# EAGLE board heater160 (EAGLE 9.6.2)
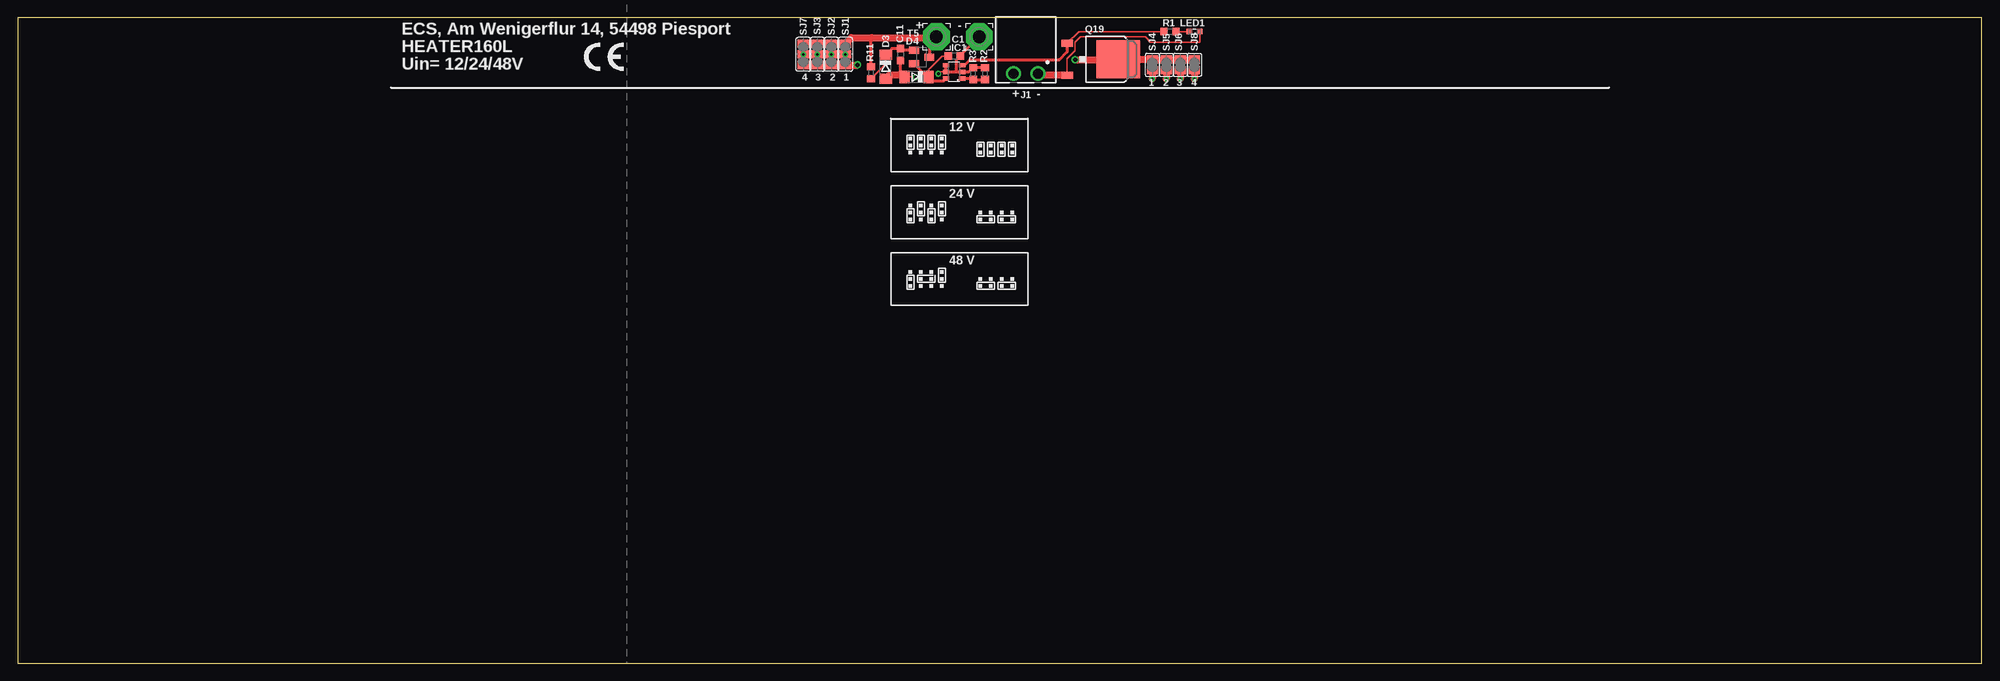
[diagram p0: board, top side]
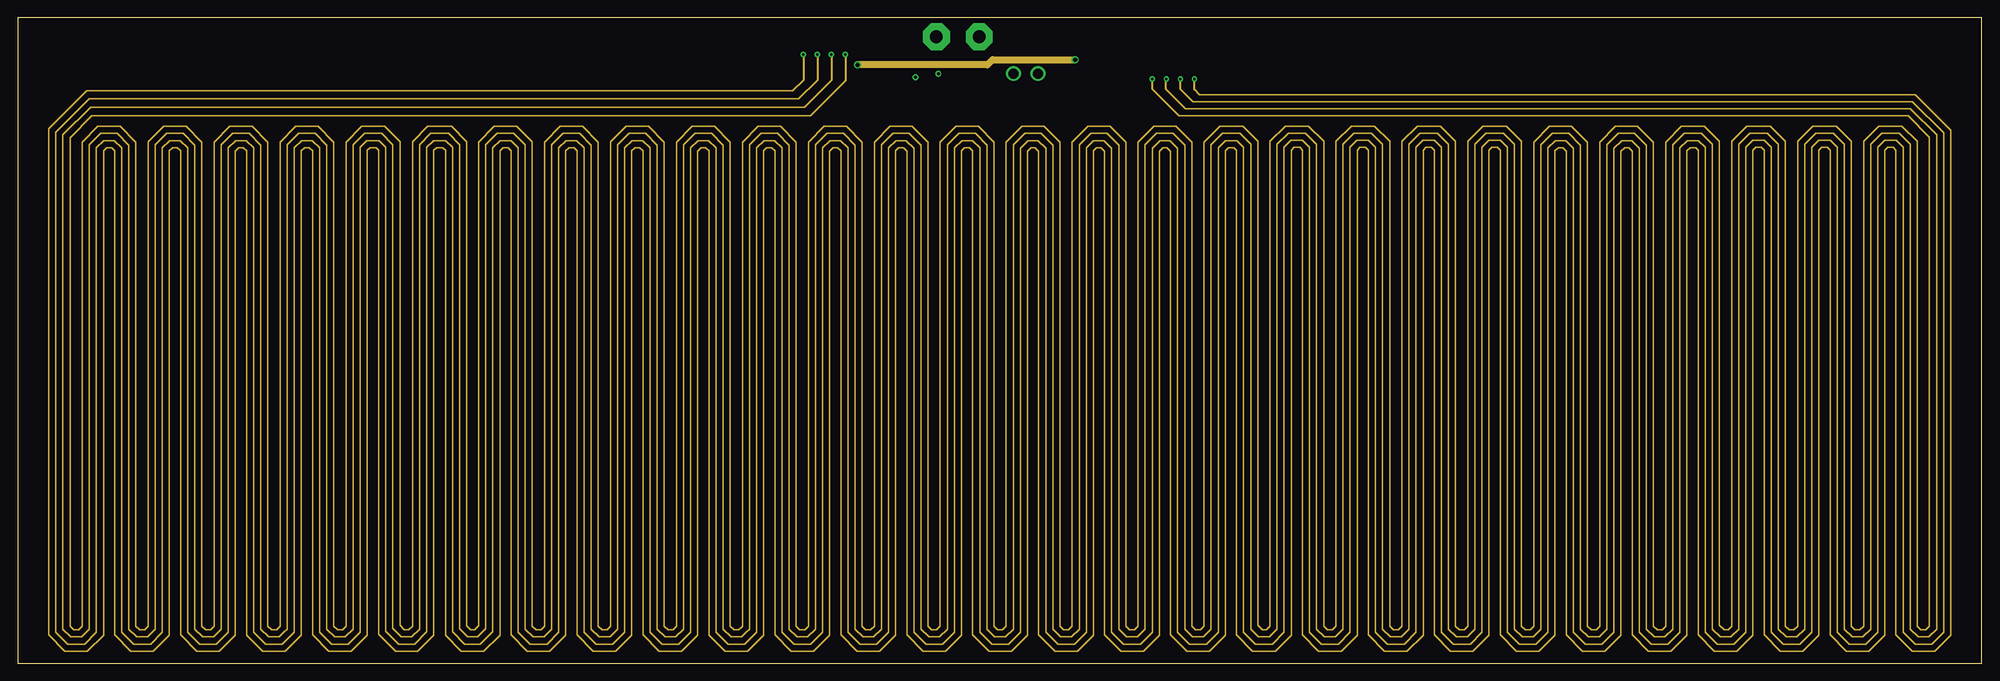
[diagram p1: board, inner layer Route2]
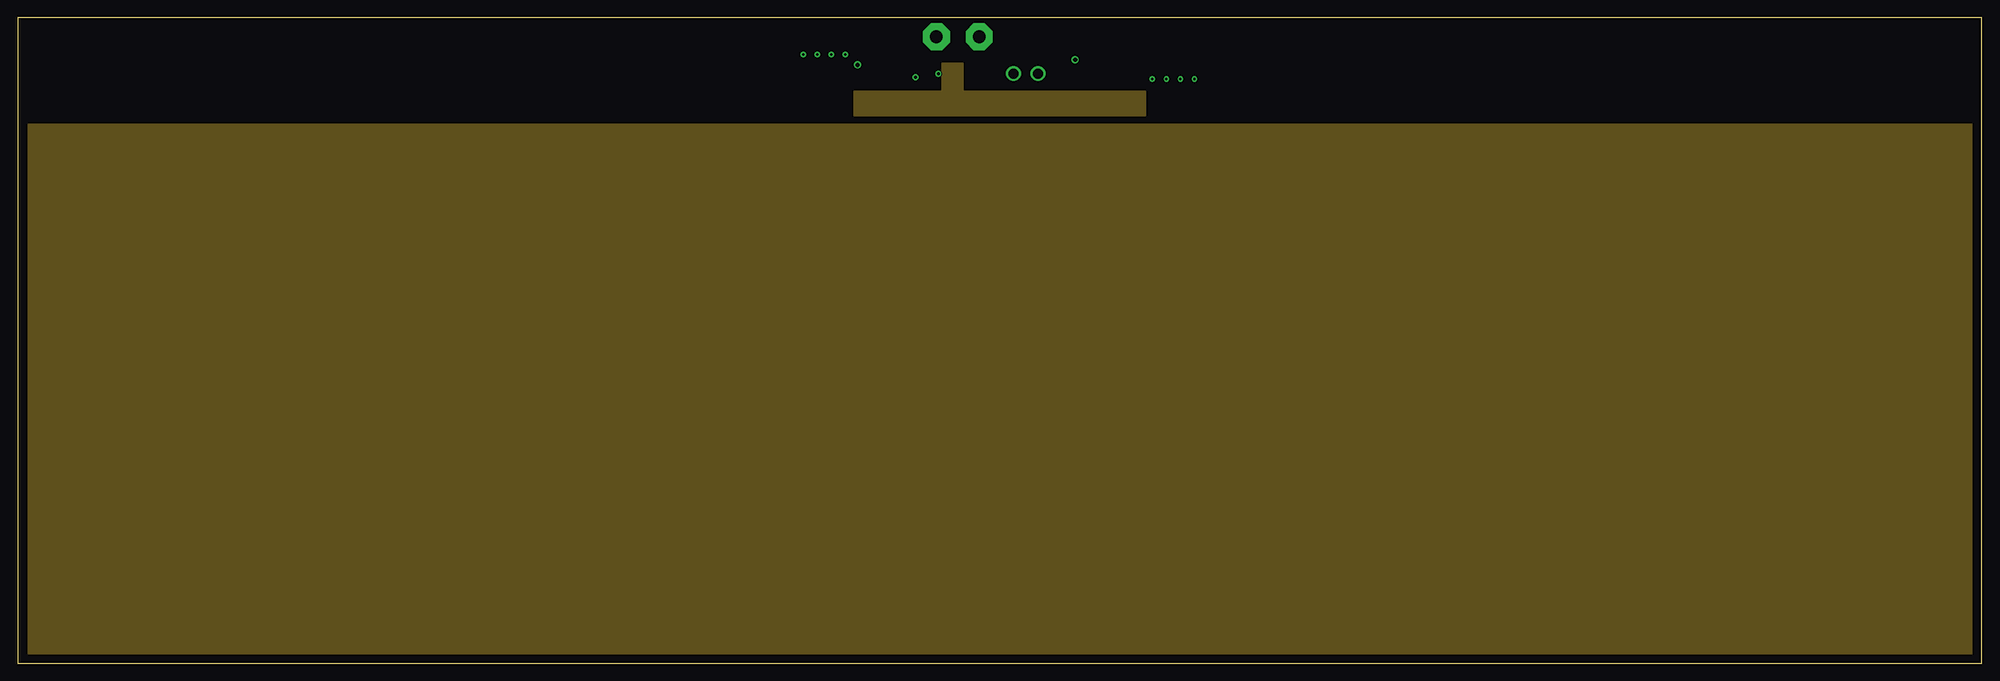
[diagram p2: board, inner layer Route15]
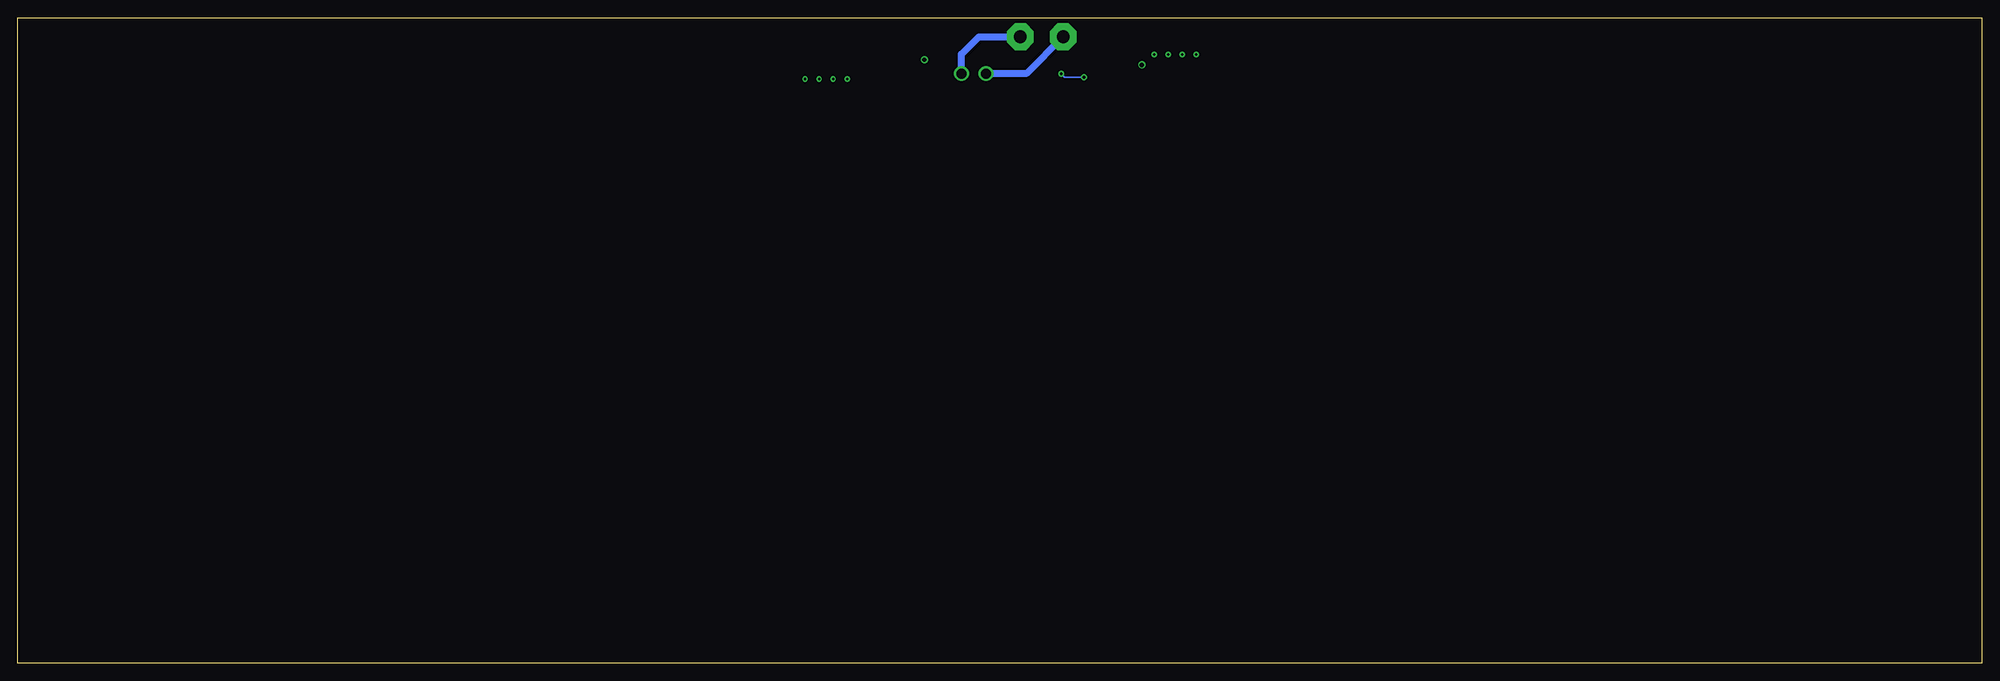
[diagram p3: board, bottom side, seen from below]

Size 280 x 92 mm. Coordinates in mm from the lower left corner, seen from the top.
Outline: 0,0 280,0 280,92 0,92 0,0
Copper layers (1+2*15+16): Top 0.035mm / dielectric 1.5mm / Route2 0.0175mm / dielectric 0.15mm / Route15 0.0175mm / dielectric 0.2mm / Bottom 0.035mm
Design rules "default *": minimum track width 6mil, minimum drill 0.35mm, track to track 6mil, track to pad 6mil, pad to pad 6mil, via to via 6mil, smd to smd 6mil, copper to edge 40mil, drill to drill 6mil, minimum pad ring 10mil, minimum via ring 8mil, stop-mask expansion 4mil, vias tented up to drill 0mil, thermal gap 10mil

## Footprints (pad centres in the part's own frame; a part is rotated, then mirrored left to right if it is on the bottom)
C0603 = smd 1.1 x 1: 1 -0.85,0; 2 0.85,0
SOD80C = smd 1.4 x 1.8: A 1.7,0; C -1.7,0
SOT23-6 = smd 0.6 x 0.9: 1 -0.95,-1.15; 2 0,-1.15; 3 0.95,-1.15; 4 0.95,1.15; 5 0,1.15; 6 -0.95,1.15
691322110002 = drill 1.4: 1 -1.75,0; 2 1.75,0
SML0603 = smd 0.8 x 0.8: A 0.75,0; C -0.75,0
3,81/1,4 = drill 1.8 pad 3.81 octagon: 1 0,0
D-PACK = smd 1 x 1.6: 1 -2.28,-4.8; 3 2.28,-4.8 | smd 5.4 x 6.2: 4 0,2.5
R0603 = smd 1 x 1.1: 1 -0.85,0; 2 0.85,0
SJ_2 = smd 1.168 x 1.6: 1 -1.524,0; 2 0,0; 3 1.524,0
SJ = smd 1.168 x 1.6: 1 -0.762,0; 2 0.762,0
SOT23-BEC = smd 1 x 1.4: B -0.95,-1.1; C 0,1.1; E 0.95,-1.1

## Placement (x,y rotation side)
C1  100n  [C0603]  133.52,86.52 0 top
C11  100n  [C0603]  125.85,86.73 270 top
D3  5V6  [SOD80C]  123.75,85 270 top
D4  5V1  [SOD80C]  128.13,83.55 180 top
IC1  MCP9510H  [SOT23-6]  133.5,84.25 90 top
J1  [691322110002]  143.71,84.01 180 top
LED1  [SML0603]  167.75,90 180 top
PAD1  [3,81/1,4]  130.97,89.26 0 top
PAD2  [3,81/1,4]  137.07,89.26 0 top
Q19  IRLR3110Z  [D-PACK]  154.41,86.05 270 top
R1  10k  [R0603]  164.25,90 180 top
R2  82k  [R0603]  137.89,84.02 270 top
R3  2M2  [R0603]  136.22,84.02 270 top
R11  100k  [R0603]  121.65,84.12 90 top
SJ1  [SJ_2]  118,86.75 90 top
SJ2  [SJ_2]  116,86.75 90 top
SJ3  [SJ_2]  114,86.75 90 top
SJ4  [SJ]  161.75,85.25 270 top
SJ5  [SJ]  163.75,85.25 270 top
SJ6  [SJ]  165.75,85.25 270 top
SJ7  [SJ_2]  112,86.75 90 top
SJ8  [SJ]  167.75,85.25 270 top
T5  BSR19A  [SOT23-BEC]  128.86,86.36 270 top
U$1  [CE-4MM]  80.75,84.38 0 top

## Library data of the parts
C1 C11 = rcl; PARTNO: C067; SPICEPREFIX: C
D3 = diode; PARTNO: D013
D4 = diode; PARTNO: D012
IC1 = mcp9509; PARTNO: IC333
J1 = Wurth_Connectors_WR-TBL Pluggable Connector; DATASHEET-URL: https://www.we-online.com/catalog/datasheet/691322110002.pdf; IR-UL: 10A; IR-VDE: 10.5A; MOUNT: THT; PART-NUMBER: 691322110002; PARTNO: CON212; PINS: 2; PITCH: 3.5mm; TYPE: Horizontal; WORKING-VOLTAGE-UL: 300V (AC); WORKING-VOLTAGE-VDE: 300V (AC)
LED1 = led; PARTNO: D078
PAD1 PAD2 = wirepad
Q19 = IRFR2607; PARTNO: T086
R1 = rcl; PARTNO: R221; SPICEPREFIX: R
R2 = rcl; PARTNO: R243; SPICEPREFIX: R
R3 = rcl; PARTNO: R277; SPICEPREFIX: R
R11 = rcl; PARTNO: R245; SPICEPREFIX: R
SJ1-SJ8 = jumper
T5 = transistor-neu-to92; PARTNO: T056
U$1 = logo

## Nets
+UB: J1.2 PAD1.1 R11.2 SJ1.3 SJ2.3 SJ3.3 SJ7.3 T5.C
GND: C1.2 C11.2 D3.A D4.A IC1.2 IC1.4 IC1.5 J1.1 LED1.C PAD2.1 Q19.3 R2.1 R3.1
N$1: IC1.3 Q19.1 R1.2
N$2: SJ1.2 SJ4.2
N$3: C11.1 D3.C R11.1 T5.B
N$4: IC1.1 R2.2 R3.2
N$5: C1.1 D4.C IC1.6 T5.E
N$6: LED1.A R1.1
N$7: SJ2.2 SJ5.2
N$8: SJ3.2 SJ6.2
N$9: SJ7.2 SJ8.2
N$11: Q19.4 SJ1.1 SJ2.1 SJ3.1 SJ4.1 SJ5.1 SJ6.1 SJ7.1 SJ8.1

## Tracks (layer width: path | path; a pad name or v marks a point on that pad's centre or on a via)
+UB
  Top 0.406: T5.C 130,86.4 130,88.29 130.85,89.14 PAD1.1 | R11.2 121.65,89.05 121.75,89.14
  Top 1.016: SJ7.3 SJ3.3 SJ2.3 SJ1.3 118.87,89.14 121.75,89.14 130.85,89.14
  Bottom 1.016: PAD1.1 136.22,84.01 J1.2
GND  (via drill 0.4)
  Top 0.2: LED1.C 168.5,88.5 161.5,88.5 160.75,89.25 151.5,89.25 150.75,88.5 150.75,87.25 149.61,86.11 Q19.3 | D4.A 127.95,83.55 v128,83.5 | v131.25,84 131.5,84.25 IC1.5
  Top 0.406: D4.A 125.85,84.13 C11.2 | 133.81,84.25 IC1.2 135.6,84.25 R3.1 R2.1 | 133.81,84.25 133.81,85.96 C1.2 134.37,86.56 PAD2.1 | IC1.4 IC1.5 133.81,84.25
  Top 1.016: D3.A 124.2,83.75 126.23,83.75 D4.A | Q19.3 145.7,83.77 J1.1
  Bottom 0.2: v128,83.5 130.75,83.5 v131.25,84
  Bottom 1.016: J1.1 145.46,86.79 142.99,89.26 PAD2.1
N$1
  Top 0.2: Q19.1 151.28,90 R1.2
  Top 0.406: IC1.3 134.95,85.2 135.75,86 148.5,86 149.61,87.11 Q19.1
N$2  (via drill 0.35, 0.35 pad 0.21)
  Top 1.016: SJ4.2 v161.75,83.25
  Route2 0.2: 118,83.02 113.04,78 10.61,78 7.48,74.87 7.48,5.27 8.01,4.75 8.71,4.75 9.22,5.25 9.22,74.26 11.45,76.49 14.64,76.49 16.88,74.25 16.88,5.27 17.4,4.75 18.11,4.75 18.62,5.25 18.62,74.27 20.84,76.49 24.04,76.49 26.28,74.25 26.28,5.27 26.8,4.75 27.51,4.75 28.02,5.25 28.02,74.26 30.25,76.49 33.44,76.49 35.68,74.25 35.68,5.27 36.2,4.75 36.9,4.75 37.2,5.05 37.42,5.27 37.42,74.26 39.65,76.49 42.84,76.49 45.08,74.25 45.08,5.27 45.6,4.75 46.32,4.75 46.82,5.25 46.82,74.26 49.05,76.49 52.31,76.49 54.5,74.3 54.5,5.37 55.12,4.76 55.76,4.76 56.29,5.28 56.29,74.32 58.46,76.49 61.84,76.49 64.01,74.32 64.01,5.32 64.59,4.75 65.13,4.75 65.72,5.34 65.72,74.26 67.95,76.49 71.16,76.49 73.38,74.27 73.38,5.27 73.91,4.75 74.61,4.75 75.12,5.25 75.12,74.26 77.35,76.49 80.54,76.49 82.78,74.25 82.78,5.27 83.3,4.75 84.01,4.75 84.52,5.25 84.52,74.27 86.74,76.49 89.94,76.49 92.18,74.25 92.18,5.27 92.7,4.75 93.41,4.75 93.92,5.25 93.92,74.26 96.15,76.49 99.34,76.49 101.58,74.25 101.58,5.27 102.1,4.75 102.8,4.75 103.1,5.05 103.32,5.27 103.32,74.26 105.55,76.49 108.74,76.49 110.98,74.25 110.98,5.27 111.5,4.75 112.22,4.75 112.72,5.25 112.72,74.26 114.95,76.49 118.14,76.49 120.38,74.25 120.38,5.27 120.91,4.75 121.61,4.75 122.12,5.25 122.12,74.26 124.35,76.49 127.5,76.49 129.78,74.22 129.78,5.27 130.31,4.75 131.01,4.75 131.52,5.25 131.52,74.26 133.75,76.49 136.94,76.49 139.18,74.25 139.18,5.27 139.71,4.75 140.41,4.75 140.92,5.25 140.92,74.26 143.15,76.49 146.31,76.49 148.58,74.22 148.58,5.27 149.1,4.75 149.82,4.75 150.32,5.25 150.32,74.26 152.55,76.49 155.71,76.49 157.98,74.22 157.98,5.27 158.5,4.75 159.21,4.75 159.72,5.25 159.72,74.26 161.95,76.49 165.1,76.49 167.38,74.22 167.38,5.27 167.91,4.75 168.61,4.75 169.12,5.25 169.12,74.26 171.35,76.49 174.64,76.49 176.78,74.36 176.78,5.42 177.45,4.75 178.01,4.75 178.52,5.25 178.52,74.36 180.69,76.53 184,76.53 186.18,74.36 186.18,5.27 186.71,4.75 187.41,4.75 187.92,5.25 187.92,74.36 190.09,76.53 193.41,76.53 195.58,74.36 195.58,5.27 196.1,4.75 196.81,4.75 197.32,5.25 197.32,74.36 199.5,76.53 202.81,76.53 204.98,74.36 204.98,5.27 205.5,4.75 206.21,4.75 206.72,5.25 206.72,74.36 208.9,76.53 212.21,76.53 214.38,74.36 214.38,5.27 214.91,4.75 215.61,4.75 216.12,5.25 216.12,74.26 218.35,76.49 221.5,76.49 223.78,74.22 223.78,5.27 224.31,4.75 225.01,4.75 225.52,5.25 225.52,74.26 227.75,76.49 230.91,76.49 233.18,74.22 233.18,5.27 233.71,4.75 234.41,4.75 234.92,5.25 234.92,74.26 237.15,76.49 240.44,76.49 242.58,74.36 242.58,5.42 243.25,4.75 243.81,4.75 244.32,5.25 244.32,74.36 246.5,76.53 249.81,76.53 251.98,74.36 251.98,5.27 252.5,4.75 253.21,4.75 253.72,5.25 253.72,74.36 255.9,76.53 259.2,76.53 261.38,74.36 261.38,5.27 261.9,4.75 262.61,4.75 263.12,5.25 263.12,74.36 265.3,76.53 268.61,76.53 270.78,74.36 270.78,5.27 271.31,4.75 272.01,4.75 272.52,5.25 272.52,74.95 269.48,78 165.55,78 161.75,81.8
  Route2 0.254: SJ1.2 118,83.02 | 161.75,81.8 v161.75,83.25
  other vias: 118,86.75
N$3
  Top 0.2: R11.1 123.75,85.37 D3.C
  Top 0.406: D3.C 124.63,87.58 C11.1 126.12,87.31 T5.B
N$4
  Top 0.406: IC1.1 136.22,83.3 R3.2 R2.2
N$5
  Top 0.2: C1.1 132.65,86.5 131.75,86.5 129.83,84.58 D4.C
  Top 0.406: T5.E 129.62,83.55 D4.C 130.08,83.3 130.2,83.3 130.5,83 132.02,83 IC1.6
N$6
  Top 0.2: R1.1 LED1.A
N$7  (via drill 0.35, 0.35 pad 0.21)
  Top 1.016: SJ5.2 v163.75,83.25
  Route2 0.2: 116,83.05 112.15,79.2 10.4,79.2 6.47,75.27 6.47,4.85 7.59,3.73 9.13,3.73 10.23,4.84 10.23,73.84 11.87,75.48 14.23,75.48 15.87,73.84 15.87,4.85 16.99,3.74 18.53,3.74 19.63,4.84 19.63,73.85 21.26,75.48 23.62,75.48 25.27,73.84 25.27,4.85 26.39,3.73 27.93,3.73 29.03,4.84 29.03,73.84 30.67,75.48 33.02,75.48 34.67,73.84 34.67,4.85 35.78,3.73 37.32,3.73 37.97,4.38 38.43,4.85 38.43,73.84 40.07,75.48 42.42,75.48 44.07,73.84 44.07,4.85 45.19,3.73 46.73,3.73 47.83,4.84 47.83,73.84 49.47,75.48 51.91,75.48 53.49,73.9 53.49,4.95 54.7,3.75 56.18,3.75 57.3,4.86 57.3,73.9 58.88,75.48 61.42,75.48 63.01,73.9 63.01,4.9 64.17,3.73 65.55,3.73 66.73,4.92 66.73,73.84 68.37,75.48 70.74,75.48 72.37,73.85 72.37,4.85 73.49,3.73 75.03,3.73 76.13,4.84 76.13,73.84 77.77,75.48 80.13,75.48 81.77,73.84 81.77,4.85 82.89,3.74 84.43,3.74 85.53,4.84 85.53,73.85 87.16,75.48 89.52,75.48 91.17,73.84 91.17,4.85 92.29,3.73 93.83,3.73 94.93,4.84 94.93,73.84 96.57,75.48 98.92,75.48 100.57,73.84 100.57,4.85 101.68,3.73 103.22,3.73 103.87,4.38 104.33,4.85 104.33,73.84 105.97,75.48 108.32,75.48 109.97,73.84 109.97,4.85 111.09,3.73 112.63,3.73 113.73,4.84 113.73,73.84 115.37,75.48 117.72,75.48 119.37,73.84 119.37,4.85 120.49,3.73 122.03,3.73 123.13,4.84 123.13,73.84 124.77,75.48 127.09,75.48 128.77,73.8 128.77,4.85 129.89,3.73 131.43,3.73 132.53,4.84 132.53,73.84 134.17,75.48 136.52,75.48 138.17,73.84 138.17,4.85 139.29,3.73 140.83,3.73 141.93,4.84 141.93,73.84 143.57,75.48 145.89,75.48 147.57,73.8 147.57,4.85 148.69,3.73 150.23,3.73 151.33,4.84 151.33,73.84 152.97,75.48 155.29,75.48 156.97,73.8 156.97,4.85 158.09,3.73 159.63,3.73 160.73,4.84 160.73,73.84 162.37,75.48 164.69,75.48 166.37,73.8 166.37,4.85 167.49,3.73 169.03,3.73 170.13,4.84 170.13,73.84 171.77,75.48 174.22,75.48 175.77,73.94 175.77,4.85 176.89,3.73 178.43,3.73 179.53,4.84 179.53,73.94 181.11,75.52 183.59,75.52 185.17,73.94 185.17,4.85 186.29,3.73 187.83,3.73 188.93,4.84 188.93,73.94 190.51,75.52 192.99,75.52 194.57,73.94 194.57,4.85 195.69,3.73 197.23,3.73 198.33,4.84 198.33,73.94 199.91,75.52 202.39,75.52 203.97,73.94 203.97,4.85 205.09,3.73 206.63,3.73 207.73,4.84 207.73,73.94 209.31,75.52 211.79,75.52 213.37,73.94 213.37,4.85 214.49,3.73 216.03,3.73 217.13,4.84 217.13,73.84 218.77,75.48 221.09,75.48 222.77,73.8 222.77,4.85 223.89,3.73 225.43,3.73 226.53,4.84 226.53,73.84 228.17,75.48 230.49,75.48 232.17,73.8 232.17,4.85 233.29,3.73 234.83,3.73 235.93,4.84 235.93,73.84 237.57,75.48 240.02,75.48 241.57,73.94 241.57,4.85 242.69,3.73 244.23,3.73 245.33,4.84 245.33,73.94 246.91,75.52 249.39,75.52 250.97,73.94 250.97,4.85 252.09,3.73 253.63,3.73 254.73,4.84 254.73,73.94 256.31,75.52 258.79,75.52 260.37,73.94 260.37,4.85 261.49,3.73 263.03,3.73 264.13,4.84 264.13,73.94 265.71,75.52 268.19,75.52 269.77,73.94 269.77,4.85 270.89,3.73 272.43,3.73 273.53,4.84 273.53,75.27 269.79,79.01 166.47,79.01 163.71,81.76
  Route2 0.254: SJ2.2 116,83.05 | 163.71,81.76 163.71,83.21
  Route2 0.4: 163.71,83.21 v163.75,83.25
  other vias: 116,86.75
N$8  (via drill 0.35, 0.35 pad 0.21)
  Top 1.016: SJ6.2 v165.75,83.25
  Route2 0.2: 114,83.05 111.35,80.4 10.2,80.4 5.46,75.66 5.46,4.43 7.17,2.73 9.55,2.73 11.24,4.42 11.24,73.43 12.28,74.47 13.81,74.47 14.86,73.42 14.86,4.43 16.57,2.73 18.95,2.73 20.64,4.42 20.64,73.44 21.68,74.47 23.21,74.47 24.26,73.42 24.26,4.43 25.97,2.73 28.35,2.73 30.04,4.42 30.04,73.43 31.09,74.47 32.61,74.47 33.66,73.42 33.66,4.43 35.37,2.73 37.73,2.73 39.44,4.43 39.44,73.43 40.49,74.47 42.01,74.47 43.06,73.42 43.06,4.43 44.77,2.73 47.15,2.73 48.84,4.42 48.84,73.53 49.79,74.47 51.51,74.47 52.48,73.5 52.48,4.53 54.29,2.73 56.59,2.73 58.3,4.45 58.3,73.48 59.29,74.47 61.01,74.47 61.99,73.48 61.99,4.48 63.75,2.73 65.97,2.73 67.74,4.5 67.74,73.43 68.79,74.47 70.32,74.47 71.36,73.44 71.36,4.43 73.07,2.73 75.45,2.73 77.14,4.42 77.14,73.43 78.18,74.47 79.71,74.47 80.76,73.42 80.76,4.43 82.47,2.73 84.85,2.73 86.54,4.42 86.54,73.44 87.58,74.47 89.11,74.47 90.16,73.42 90.16,4.43 91.87,2.73 94.25,2.73 95.94,4.42 95.94,73.43 96.99,74.47 98.51,74.47 99.56,73.42 99.56,4.43 101.27,2.73 103.63,2.73 105.34,4.43 105.34,73.43 106.39,74.47 107.91,74.47 108.96,73.42 108.96,4.43 110.67,2.73 113.05,2.73 114.74,4.42 114.74,73.43 115.79,74.47 117.31,74.47 118.36,73.42 118.36,4.43 120.07,2.73 122.45,2.73 124.14,4.42 124.14,73.43 125.19,74.47 126.67,74.47 127.76,73.38 127.76,4.43 129.47,2.73 131.85,2.73 133.54,4.42 133.54,73.43 134.59,74.47 136.11,74.47 137.16,73.42 137.16,4.43 138.87,2.73 141.25,2.73 142.94,4.42 142.94,73.36 144.05,74.47 145.47,74.47 146.56,73.38 146.56,4.43 148.27,2.73 150.65,2.73 152.34,4.42 152.34,73.43 153.39,74.47 154.87,74.47 155.96,73.38 155.96,4.43 157.67,2.73 160.05,2.73 161.74,4.42 161.74,73.36 162.85,74.47 164.27,74.47 165.36,73.38 165.36,4.43 167.07,2.73 169.45,2.73 171.14,4.42 171.14,73.43 172.19,74.47 173.81,74.47 174.76,73.52 174.76,4.43 176.47,2.73 178.85,2.73 180.54,4.42 180.54,73.52 181.53,74.51 183.17,74.51 184.16,73.52 184.16,4.43 185.87,2.73 188.25,2.73 189.94,4.42 189.94,73.52 190.93,74.51 192.57,74.51 193.56,73.52 193.56,4.43 195.27,2.73 197.65,2.73 199.34,4.42 199.34,73.52 200.33,74.51 201.97,74.51 202.96,73.52 202.96,4.43 204.67,2.73 207.05,2.73 208.74,4.42 208.74,73.52 209.73,74.51 211.37,74.51 212.36,73.52 212.36,4.43 214.07,2.73 216.45,2.73 218.14,4.42 218.14,73.43 219.19,74.47 220.67,74.47 221.76,73.38 221.76,4.43 223.47,2.73 225.85,2.73 227.54,4.42 227.54,73.36 228.65,74.47 230.07,74.47 231.16,73.38 231.16,4.43 232.87,2.73 235.25,2.73 236.94,4.42 236.94,73.43 237.99,74.47 239.61,74.47 240.56,73.52 240.56,4.43 242.27,2.73 244.65,2.73 246.34,4.42 246.34,73.52 247.33,74.51 248.97,74.51 249.96,73.52 249.96,4.43 251.67,2.73 254.05,2.73 255.74,4.42 255.74,73.52 256.73,74.51 258.37,74.51 259.36,73.52 259.36,4.43 261.07,2.73 263.45,2.73 265.14,4.42 265.14,73.52 266.13,74.51 267.77,74.51 268.76,73.52 268.76,4.43 270.47,2.73 272.85,2.73 274.54,4.42 274.54,75.56 270.08,80.02 167.53,80.02 165.75,81.8
  Route2 0.254: SJ3.2 114,83.05 | 165.75,81.8 v165.75,83.25
  other vias: 114,86.75
N$9  (via drill 0.35, 0.35 pad 0.21)
  Top 1.016: SJ8.2 v167.75,83.25
  Route2 0.2: 112,83.05 110.5,81.55 9.85,81.55 4.45,76.15 4.45,4.02 6.75,1.72 9.97,1.72 12.25,4 12.25,73.01 12.7,73.45 13.4,73.45 13.85,73 13.85,4.02 16.15,1.72 19.37,1.72 21.65,4 21.65,73.02 22.09,73.46 22.79,73.46 23.25,73 23.25,4.02 25.55,1.72 28.77,1.72 31.05,4 31.05,72.96 31.55,73.46 32.19,73.46 32.65,73 32.65,4 34.95,1.72 38.15,1.72 40.45,4 40.45,73.01 40.9,73.45 41.6,73.45 42.05,73 42.05,4.02 44.35,1.72 47.57,1.72 49.85,4 49.85,73.06 50.25,73.46 51.11,73.46 51.48,73.1 51.48,4.12 53.88,1.72 57.04,1.72 59.31,3.99 59.31,73.06 59.71,73.46 60.59,73.46 60.99,73.06 60.99,3.98 63.25,1.72 66.47,1.72 68.75,4 68.75,73.01 69.2,73.45 69.91,73.45 70.35,73.02 70.35,4.02 72.65,1.72 75.87,1.72 78.15,4 78.15,73.01 78.6,73.45 79.3,73.45 79.75,73 79.75,4.02 82.05,1.72 85.27,1.72 87.55,4 87.55,73.02 87.99,73.46 88.69,73.46 89.15,73 89.15,4.02 91.45,1.72 94.67,1.72 96.95,4 96.95,72.96 97.45,73.46 98.09,73.46 98.55,73 98.55,4 100.85,1.72 104.05,1.72 106.35,4 106.35,73.01 106.8,73.45 107.5,73.45 107.95,73 107.95,4.02 110.25,1.72 113.47,1.72 115.75,4 115.75,72.96 116.25,73.46 116.89,73.46 117.35,73 117.35,4.02 119.65,1.72 122.87,1.72 125.15,4 125.15,73.01 125.61,73.46 126.25,73.46 126.75,72.96 126.75,4.02 129.05,1.72 132.27,1.72 134.55,4 134.55,73.01 135,73.46 135.69,73.46 136.15,73 136.15,4.02 138.45,1.72 141.67,1.72 143.95,4 143.95,72.94 144.47,73.46 145.05,73.46 145.55,72.96 145.55,4.02 147.85,1.72 151.07,1.72 153.35,4 153.35,73.01 153.81,73.46 154.45,73.46 154.95,72.96 154.95,4.02 157.25,1.72 160.47,1.72 162.75,4 162.75,72.94 163.27,73.46 163.85,73.46 164.35,72.96 164.35,4.02 166.65,1.72 169.87,1.72 172.15,4 172.15,73.01 172.6,73.46 173.39,73.46 173.75,73.1 173.75,4.02 176.05,1.72 179.27,1.72 181.55,4 181.55,73.1 181.95,73.5 182.75,73.5 183.15,73.1 183.15,4.02 185.45,1.72 188.67,1.72 190.95,4 190.95,73.1 191.35,73.5 192.15,73.5 192.55,73.1 192.55,4.02 194.85,1.72 198.07,1.72 200.35,4 200.35,73.1 200.75,73.5 201.55,73.5 201.95,73.1 201.95,4.02 204.25,1.72 207.47,1.72 209.75,4 209.75,73.1 210.15,73.5 210.95,73.5 211.35,73.1 211.35,4.02 213.65,1.72 216.87,1.72 219.15,4 219.15,73.01 219.6,73.46 220.25,73.46 220.75,72.96 220.75,4.02 223.05,1.72 226.27,1.72 228.55,4 228.55,72.94 229.07,73.46 229.65,73.46 230.15,72.96 230.15,4.02 232.45,1.72 235.67,1.72 237.95,4 237.95,73.01 238.41,73.46 239.19,73.46 239.55,73.1 239.55,4.02 241.85,1.72 245.07,1.72 247.35,4 247.35,73.1 247.75,73.5 248.55,73.5 248.95,73.1 248.95,4.02 251.25,1.72 254.47,1.72 256.75,4 256.75,73.1 257.15,73.5 257.95,73.5 258.35,73.1 258.35,4.02 260.65,1.72 263.87,1.72 266.15,4 266.15,73.1 266.55,73.5 267.35,73.5 267.75,73.1 267.75,4.02 270.05,1.72 273.27,1.72 275.55,4 275.55,75.95 270.47,81.03 168.47,81.03 167.75,81.75
  Route2 0.254: SJ7.2 112,83.05 | 167.75,81.75 v167.75,83.25
  other vias: 112,86.75
N$10
  pour Route15: 131.75,85.5 131.75,81.5 119.25,81.5 119.25,78 160.75,78 160.75,81.5 134.75,81.5 134.75,85.5
N$11  (via drill 0.6)
  Top 1.016: SJ7.1 SJ3.1 SJ2.1 SJ1.1 119.73,85.23 v119.75,85.25 | SJ8.1 SJ6.1 SJ5.1 SJ4.1 157.9,86.01 156.91,87 Q19.4 156.86,86 v150.75,86
  Route2 1.016: v119.75,85.25 138.25,85.25 139,86 v150.75,86
N$12
  pour Route15: 278.55,76.75 1.55,76.75 1.55,1.4 278.55,1.4

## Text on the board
tPlace: ECS, Am Wenigerflur 14, 54498 Piesport | + | - | HEATER160L | Uin= 12/24/48V | 4 | 3 | 2 | 1 | 1 | 2 | 3 | 4 | + | - | 12 V | 24 V | 48 V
